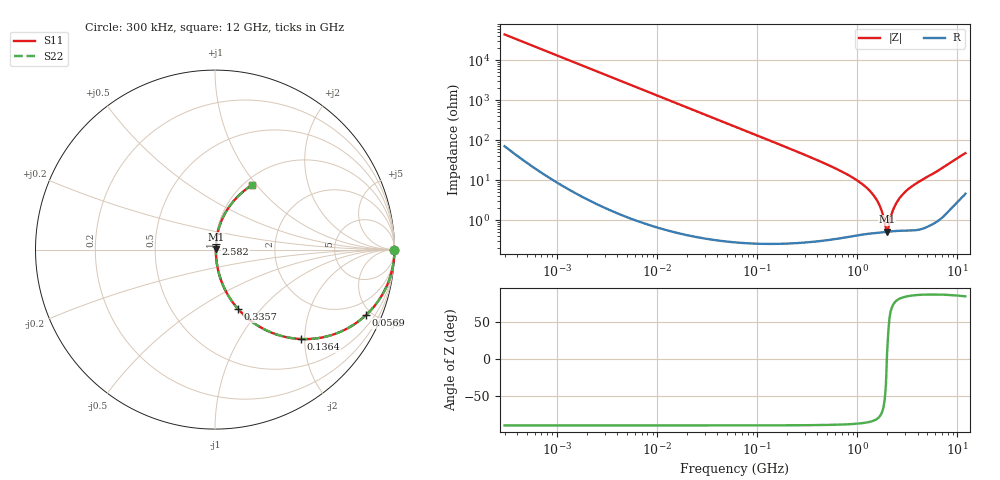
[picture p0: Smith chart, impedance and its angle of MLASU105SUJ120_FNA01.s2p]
! MLASU105SUJ120_FNA01  S-PARAMETER MODEL  ( General Type )
! Model Generated by TAIYO YUDEN Corporation (http://www.ty-top.com)
! Version 2.0
! TAIYO YUDEN Control No. 120810
! Copyright(c) 2011 TAIYO YUDEN CO.,LTD. All Rights Reserved.
! Product Description (link to TY-COMPAS)
! https://ds.yuden.co.jp/TYCOMPAS/or/detail?pn=MLASU105SUJ120JFNA01&u=M
! Products Name : Multilayer Ceramic Capacitors
! Characteristics :
!  Capacitance : 12 pF , Rated Voltage : 50V , TCC : UJ / U2J
!  Case Size : 1.0 x 0.5 / 0.039 x 0.02 [mm/inch] , Thickness : 0.5 / 0.02 [mm/inch]
!  (Conditions: Temperature = 25 degC , DC Bias Current/Voltage = 0A / 0V)
! External Node Assignments :
!  1  o---| |---o  2
! GND o---------o GND
! Frequency Range : 0.3MHz  -  12000MHz  [ 401 STEP ]
# MHz S RI R 50
! Freq[MHz].  S11 Real  S11 Imag  S21 Real  S21 Imag  S12 Real  S12 Imag  S22 Real  S22 Imag
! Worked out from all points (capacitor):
!   401 points, 300 kHz to 12 GHz, reference 50 ohm
!   read as one part in series: C = 12.1 pF near 316.3 kHz
!   lowest |Z| = 515 mohm at 1.981 GHz (marker M1)
!   series resonance near 1.973 GHz, so ESL is about 540 pH
!   S11 on the Smith chart (normalised r, x): 300 kHz: open; 56.9 MHz: 1.01, -4.63; 136.4 MHz: 1.01, -1.92; 335.7 MHz: 1.01, -0.76; 2.582 GHz: 1.01, +0.07; 12 GHz: 1.09, +0.94
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0.3  1 -0.00227  8.84e-06 0.00227  8.84e-06 0.00227  1 -0.00227
1.769972  0.9998 -0.0134  0.000187 0.0134  0.000187 0.0134  0.9998 -0.0134
10.44266  0.9937 -0.0787  0.00627 0.0787  0.00627 0.0787  0.9937 -0.0787
29.34352  0.9527 -0.212  0.0473 0.212  0.0473 0.212  0.9527 -0.212
56.90376  0.8425 -0.3636  0.1575 0.3636  0.1575 0.3636  0.8425 -0.3636
60  0.8279 -0.3768  0.1721 0.3768  0.1721 0.3768  0.8279 -0.3768
136.3989  0.4809 -0.4983  0.5191 0.4983  0.5191 0.4983  0.4809 -0.4983
335.7268  0.1289 -0.3314  0.8711 0.3314  0.8711 0.3314  0.1289 -0.3314
353.9943  0.1171 -0.3175  0.8829 0.3175  0.8829 0.3175  0.1171 -0.3175
763.2128  0.0247 -0.143  0.9753 0.143  0.9753 0.143  0.0247 -0.143
1229.528  0.00878 -0.0651  0.9912 0.0651  0.9912 0.0651  0.00878 -0.0651
1602.47  0.00564 -0.0281  0.9944 0.0281  0.9944 0.0281  0.00564 -0.0281
1735.023  0.00524 -0.0175  0.9948 0.0175  0.9948 0.0175  0.00524 -0.0175
1878.541  0.00506 -0.00698  0.9949 0.00698  0.9949 0.00698  0.00506 -0.00698
1980.756  0.00508 0.000637  0.9949 -0.000637  0.9949 -0.000637  0.00508 0.000637
2088.533  0.00522 0.0071  0.9948 -0.0071  0.9948 -0.0071  0.00522 0.0071
2261.293  0.00556 0.0165  0.9944 -0.0165  0.9944 -0.0165  0.00556 0.0165
2581.562  0.00646 0.0322  0.9935 -0.0322  0.9935 -0.0322  0.00646 0.0322
3026.31  0.00812 0.0513  0.9919 -0.0513  0.9919 -0.0513  0.00812 0.0513
3740.715  0.0116 0.077  0.9884 -0.077  0.9884 -0.077  0.0116 0.077
7254.098  0.0538 0.198  0.9462 -0.198  0.9462 -0.198  0.0538 0.198
12000  0.2059 0.3586  0.7941 -0.3586  0.7941 -0.3586  0.2059 0.3586
